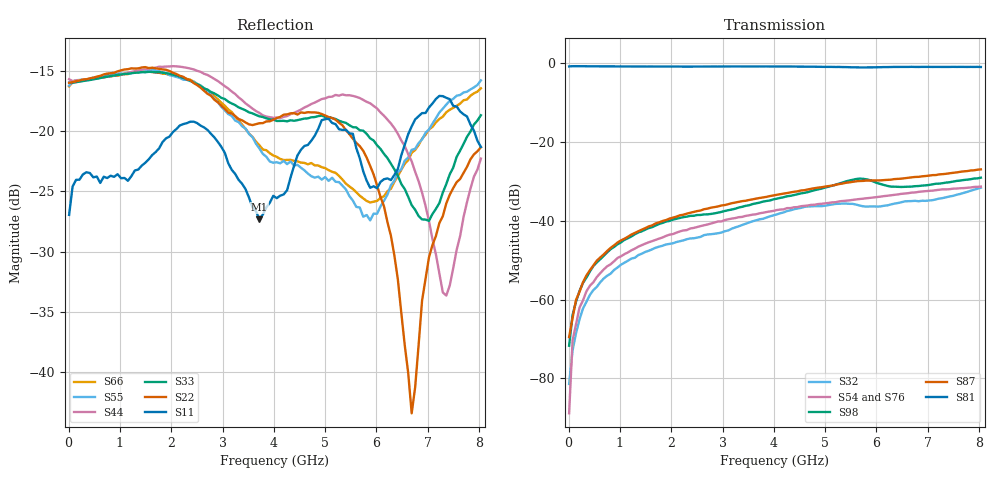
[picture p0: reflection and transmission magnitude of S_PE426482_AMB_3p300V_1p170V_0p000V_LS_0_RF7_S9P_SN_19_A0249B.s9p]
! Device ID: PE426482
! File Path: z:\PE426482\Final Char Data\room\AMB\3p300\LS_0_RF7\PE426482_AMB_3p300V_1p170V_0p000V_LS_0_RF7_S9P_SN_19_A0249B.s9p
! Serial: 19
! Lot: A0249B
! Temp: AMB
! VDD: 3.300
! VSS: 0.000
! Control_Hi: 1.170
! Control_Lo: 0.000
! Logic State: LS_0_RF7
! Port 1:
! Port 2:
! Port 3:
! Port 4:
! Port 5:
! Port 6:
! Port 7:
! Port 8:
! Port 9:
! ThroughPath:1-8
! IDD: 0.0001087762
! ISS/IDD2: -1.43e-008
! IDMM3/IDD3: -2.332e-007
! Comment:
#  Hz  S  RI  R  50
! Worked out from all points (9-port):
!   120 points, 10 MHz to 8.037 GHz, reference 50 ohm
!   strongest paths, dB at 10 MHz, 2.034 GHz, 4.057 GHz, 6.08 GHz, 8.037 GHz:
!     S81: -0.9, -0.9, -0.9, -1.0, -1.0
!     S87: -69.5, -39.2, -33.4, -29.8, -27.0
!     S98: -71.7, -39.7, -34.4, -30.7, -29.1
!     S54: -88.9, -43.4, -37.3, -33.9, -31.3
!     S76: -81.0, -43.2, -37.4, -33.7, -31.3
!     S32: -81.4, -45.7, -38.4, -36.4, -31.6
!   lowest |S11| = -27.3 dB at 3.72 GHz (marker M1), VSWR 1.09, Z = 54.5 + j0.163 ohm
!   |S11| at or under -10 dB: start of sweep to end of sweep
